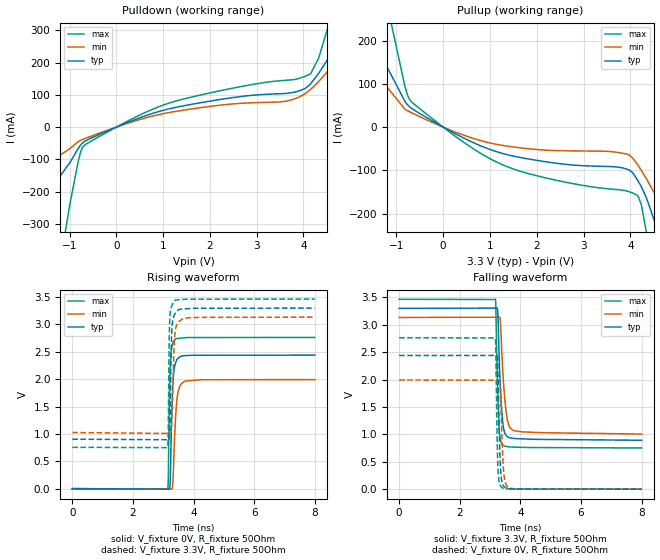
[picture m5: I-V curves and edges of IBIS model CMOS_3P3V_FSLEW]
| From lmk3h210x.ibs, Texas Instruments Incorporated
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[Model]   CMOS_3P3V_FSLEW
Model_type   Output
Polarity   Non-Inverting
Vmeas = 1.65
Vref = 1.65
Cref = 2pF
Rref = 100000
|   typ   min   max
C_comp   2.5pF   2pF   3pF
[Voltage Range]   3.3   3.135   3.465
[Temperature Range]   45   125   -40
[Pullup Reference]   3.3   3.135   3.465
[Pulldown Reference]   -0   0   0
[Power Clamp Reference]   3.3   3.135   3.465
[GND Clamp Reference]   0   0   0
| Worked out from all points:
|   slope of the pulldown table from 0 to 0.495 V, typ, clamps not added: 17.3 ohm
|   slope of the pullup table from 0 to 0.495 V, typ, clamps not added: 17.5 ohm
|   falling waveform, V_fixture 3.3V, R_fixture 50Ohm: 20-80 % time 115ps typ, 155ps min, 79.1ps max; typ from 3.3 V to 0.892 V
|   rising waveform, V_fixture 0V, R_fixture 50Ohm: 20-80 % time 76.4ps typ, 106ps min, 52.5ps max; typ from 0.001 V to 2.44 V
|   rising waveform, V_fixture 3.3V, R_fixture 50Ohm: 20-80 % time 48.9ps typ, 72.3ps min, 34.7ps max; typ from 0.903 V to 3.3 V
|   falling waveform, V_fixture 0V, R_fixture 50Ohm: 20-80 % time 66.9ps typ, 82.8ps min, 51ps max; typ from 2.44 V to 0 V
[Pulldown]
|   Voltage   I(typ)   I(min)   I(max)
-3.3V     -900.4mA   -530.4mA   -2.688A
-2.33V    -552.8mA   -290.6mA   -1.659A
-2.31V    -545.4mA   -312mA     -1.637A
-1.221V   -155.5mA   -88.35mA   -439.6mA
-993.3mV  -110.4mA   -67mA      -239.8mA
-735.9mV  -51.28mA   -39.19mA   -67.1mA
-260.7mV  -16.04mA   -13.19mA   -20.54mA
1.264V    61.12mA    48.7mA     80.63mA
3.759V    107.1mA    85.15mA    146.8mA
4.155V    135mA      117.4mA    165.8mA
4.778V    268.6mA    215.3mA    430.8mA
6.6V      722.3mA    542mA      1.425A
[Pullup]
|   Voltage   I(typ)   I(min)   I(max)
-3.3V     622.7mA    433.5mA    1.383A
-2.023V   315.3mA    210.4mA    700.3mA
-1.736V   250.9mA    163.9mA    550.9mA
-815.1mV  59.02mA    41.28mA    93.08mA
-537.9mV  34mA       26.09mA    45.85mA
1.403V    -64.57mA   -44.46mA   -92.89mA
3.67V     -91.69mA   -57.52mA   -144mA
4.125V    -117.3mA   -82.17mA   -156.2mA
4.343V    -163.5mA   -119.4mA   -243.1mA
4.571V    -234.3mA   -163.1mA   -428mA
5.056V    -416.7mA   -272.8mA   -947.3mA
6.6V      -993.8mA   -630.3mA   -2.645A
[Ramp]
R_load = 50
|   typ   min   max
dV/dt_r   1.46333/7.60254e-11   1.19537/1.05994e-10   1.65754/5.23847e-11
dV/dt_f   1.44363/1.14684e-10   1.27611/1.54588e-10   1.62721/7.89315e-11
[Falling Waveform]
V_fixture = 3.3V
V_fixture_min = 3.135V
V_fixture_max = 3.465V
R_fixture = 50Ohm
C_fixture = 0F
|   Time   V(typ)   V(min)   V(max)
0s        3.298V     3.132V     3.464V
3.174ns   3.303V     3.137V     3.468V
3.189ns   3.303V     3.137V     3.347V
3.249ns   3.27V      3.137V     1.793V
3.294ns   2.525V     3.137V     1.165V
3.337ns   1.892V     3.079V     913.4mV
3.447ns   1.101V     1.908V     794.2mV
3.572ns   957.8mV    1.262V     776.7mV
3.784ns   926.5mV    1.069V     767.7mV
8ns       891.9mV    1.005V     751.6mV
[Rising Waveform]
V_fixture = 0V
V_fixture_min = 0V
V_fixture_max = 0V
R_fixture = 50Ohm
C_fixture = 0F
|   Time   V(typ)   V(min)   V(max)
0s        654.7uV    5.03uV     353.8uV
3.147ns   -8.755mV   -7.289mV   -9.119mV
3.166ns   -8.814mV   -7.334mV   142.4mV
3.203ns   -7.929mV   -7.419mV   1.63V
3.239ns   283.2mV    -7.503mV   2.332V
3.311ns   1.824V     52.04mV    2.646V
3.406ns   2.298V     1.272V     2.736V
3.503ns   2.389V     1.795V     2.746V
3.744ns   2.431V     1.967V     2.758V
8ns       2.44V      1.992V     2.763V
[Rising Waveform]
V_fixture = 3.3V
V_fixture_min = 3.135V
V_fixture_max = 3.465V
R_fixture = 50Ohm
C_fixture = 0F
|   Time   V(typ)   V(min)   V(max)
0s        903mV      1.026V     755mV
3.143ns   894.8mV    1.009V     749.9mV
3.163ns   894.7mV    1.009V     955.9mV
3.195ns   908.3mV    1.009V     2.586V
3.217ns   1.087V     1.009V     3.105V
3.279ns   2.826V     1.193V     3.334V
3.35ns    3.152V     2.467V     3.416V
3.388ns   3.194V     2.836V     3.44V
3.829ns   3.289V     3.122V     3.462V
8ns       3.299V     3.134V     3.464V
[Falling Waveform]
|Gnd
V_fixture = 0V
V_fixture_min = 0V
V_fixture_max = 0V
R_fixture = 50Ohm
C_fixture = 0F
|   Time   V(typ)   V(min)   V(max)
0s        2.439V     1.992V     2.763V
3.166ns   2.438V     1.988V     2.758V
3.187ns   2.436V     1.988V     2.606V
3.226ns   2.431V     1.988V     1.106V
3.261ns   2.114V     1.988V     351.4mV
3.33ns    540.4mV    1.898V     75.82mV
3.406ns   103mV      748.2mV    23.6mV
3.482ns   39.45mV    166.5mV    10.25mV
3.662ns   6.489mV    18.75mV    3.197mV
8ns       148.9uV    5.03uV     32.68uV
